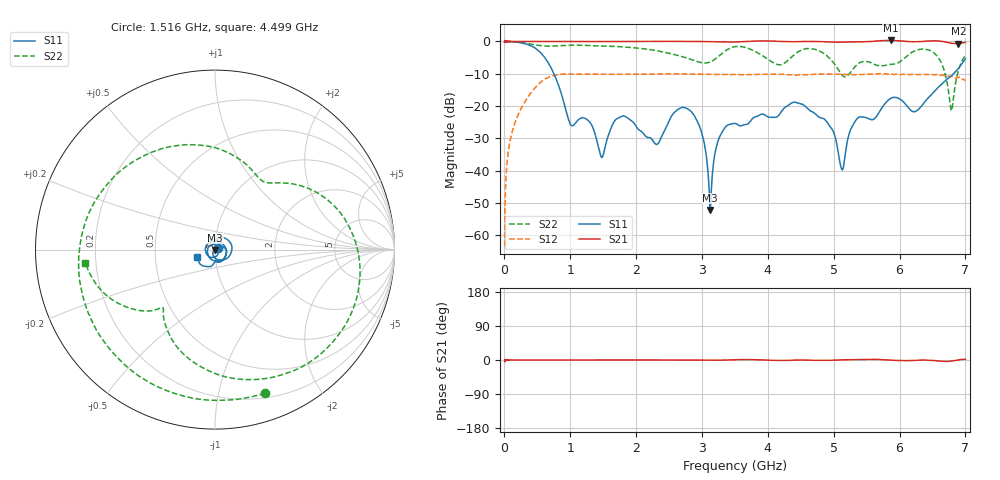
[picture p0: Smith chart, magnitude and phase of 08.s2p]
!Keysight Technologies,N5232A,MY52221221,A.10.65.11
!Date: Wednesday, October 16, 2024 11:55:38
!Correction: S11(Full 2 Port(1,4))
!S41(Full 2 Port(1,4))
!S14(Full 2 Port(1,4))
!S44(Full 2 Port(1,4))
!S2P File: Measurements: S11, S41, S14, S44:
# Hz S  RI  R 50
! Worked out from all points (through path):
!   4000 points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, 2.05 MHz to 7 GHz, reference 50 ohm
!   highest |S21| = 0.31 dB at 5.864 GHz (marker M1); lowest = -0.6 dB at 6.895 GHz (marker M2)
!   lowest |S11| = -52.1 dB at 3.126 GHz (marker M3), VSWR 1.00, Z = 50.1 - j0.24 ohm
!   |S11| at or under -10 dB: 750.9 MHz to 6.819 GHz (6.068 GHz wide, 160 % of centre)
!   |S22| runs from -21.4 to 0.0 dB; largest |S21 - S12| = 1.3
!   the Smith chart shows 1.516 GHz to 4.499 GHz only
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2049925  -0.9688 0.1509  0.9626 -0.0707  0.000122 0.00067  -0.9768 0.098
1.805423e8  -0.0367 0.9771  0.9976 -0.000563  0.0601 0.0197  -0.8137 0.5441
3.415354e8  0.8923 0.167  1 0.00109  0.0873 -0.0979  -0.429 0.8296
4.867792e8  0.2804 -0.7083  0.9996 -0.00175  -0.0806 -0.1878  -0.0491 0.8788
6.320229e8  -0.4586 -0.2591  0.9984 -0.000544  -0.2683 0.0104  0.271 0.804
1.16925e9  0.0309 0.0582  0.9974 0.000245  0.1625 -0.2662  0.8446 -0.221
1.478987e9  0.0161 0.00149  0.9968 0.000392  -0.3112 0.0126  0.3592 -0.7698
1.688978e9  0.0616 -0.00232  0.9966 0.00206  -0.0288 0.3094  -0.1286 -0.8264
2.3347e9  0.000482 0.0265  1.004 6.36e-05  -0.2873 -0.1294  -0.6398 0.3134
2.826429e9  0.0712 -0.0452  1.002 -0.00811  0.3046 0.073  0.1148 0.5169
3.125666e9  0.000616 -0.0024  0.992 -0.0113  -0.0623 -0.3031  0.3083 0.3712
3.5019e9  -0.0529 0.00982  0.9816 0.0122  -0.1246 0.28  0.7954 -0.2419
3.794137e9  0.0649 -0.0185  1.012 0.0153  0.3101 0.0116  0.0636 -0.7105
4.257868e9  -0.0206 -0.0927  0.9947 -0.0188  -0.3064 -0.0147  -0.3267 -0.3344
4.66735e9  -0.0805 0.0168  1 -0.0113  0.274 0.1403  -0.6182 0.4601
5.12758e9  0.00908 -0.00509  0.976 0.00658  -0.2743 -0.1449  0.1541 0.258
5.83455e9  -0.0835 0.0936  1.035 0.00168  0.1194 -0.289  0.4111 -0.1506
5.864299e9  -0.0772 0.1068  1.036 -0.00501  0.0576 -0.3099  0.4053 -0.1778
6.494272e9  0.00822 0.1547  1.023 -0.018  0.2715 0.1468  -0.6272 -0.3062
6.784759e9  0.2879 -0.0545  0.9415 -0.0455  -0.0149 -0.2862  -0.0858 0.00272
6.895004e9  0.0838 -0.3742  0.9287 0.00228  -0.2202 -0.1752  -0.2741 -0.2318
7e9  -0.4433 -0.3081  0.9658 0.0333  -0.2439 0.0439  -0.6079 -0.0465
